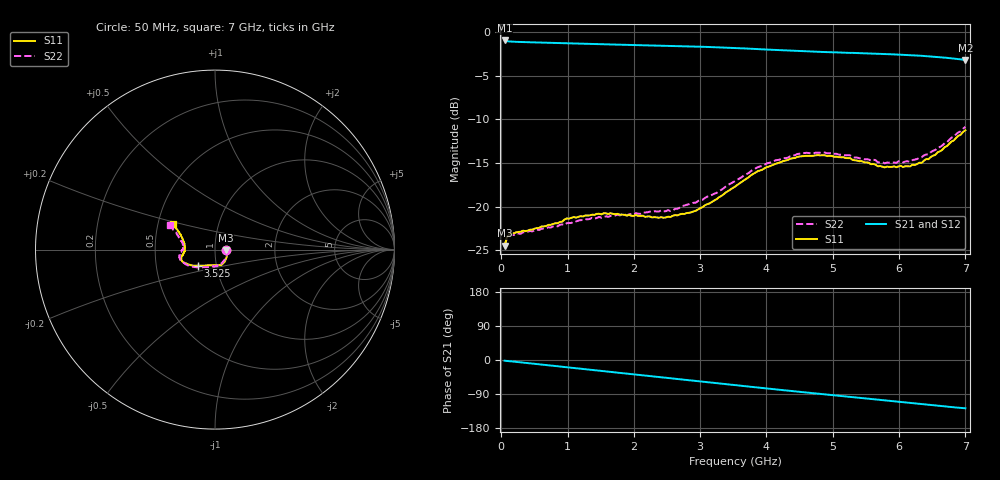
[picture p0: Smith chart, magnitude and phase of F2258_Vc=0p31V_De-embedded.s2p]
! Integrated Device Technology
! Corporate Headquarters
! 6024 Silver Creek Valley Road
! San Jose, CA 95138  USA
! Phone:  1-408-284-8200
! Toll Free:  1-800-223-1366
! Webpage:  http://www.idt.com/
! Timing and RF Division
! 515 Groton Road, Suite 102
! Westford, MA 01886-6024
! Device:  F2258
! Description: Voltage Variable RF Attenuator
! Frequency:  50.0 -  6000.00 MHz
! Package:  3x3 mm Thin QFN Plastic Package: 16 pin
! Ports:  2 RF, 2 DC
!  Pin  1  = NC
!  Pin  2  = NC
!  Pin  3  = RF2  = Port 2
!  Pin  4  = GND
!  Pin  5  = Vdd
!  Pin  6  = NC
!  Pin  7  = VCTRL
!  Pin  8  = NC
!  Pin  9  = GND
!  Pin 10  = RF1  = Port 1
!  Pin 11  = NC
!  Pin 12  = NC
!  Pin 13  = NC
!  Pin 14  = NC
!  Pin 15  = NC
!  Pin 16  = NC
! Vcntrl:  0.310 Volts
! Vdd:  +3.300 Volts
! Current:  1.086 mA
! Data:  The device was measured on a the F2258 evaluation board which has
!  individual transmission lines to the RF pins.  Data was collected
!  using a calibrated network analyzer.  The evaluation board was
!  de-embedded using a TRL calibration technique.
!  The reference plane is the edge of the package pin.
! Misc:  SN 10
!  Action Tracker AT0285
! Date Measured:  2014-12-10
! Date:  2016-01-13  MJV
! Note:
!  Integrated Device Technology supplies this data as a sample of measured
!  data at the package pin for this product.  Your particular data for this
!  product may vary.
!  Data was taken at 25 degrees C.
!  Integrated Device Technology reserves the right to change this data at anytime.
!Freq_(GHz)  S11M_(dB)  S11P_(deg)  S21M_(dB)  S21P_(deg)  S12M_(dB)  S12P_(deg)  S22M_(dB)  S22P_(deg)
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# GHz S dB R 50
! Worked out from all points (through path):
!   201 points, 50 MHz to 7 GHz, reference 50 ohm
!   highest |S21| = -0.98 dB at 50 MHz (marker M1); lowest = -3.2 dB at 7 GHz (marker M2)
!   group delay of S21, straight-line fit = 50.5 ps
!   lowest |S11| = -24.5 dB at 50 MHz (marker M3), VSWR 1.13, Z = 56.3 - j0.398 ohm
!   |S11| at or under -10 dB: start of sweep to end of sweep
!   |S22| runs from -24.5 to -10.9 dB; largest |S21 - S12| = 0.00045
!   S11 on the Smith chart (normalised r, x): 50 MHz: 1.13, -0.01; 3.525 GHz: 0.82, -0.15; 7 GHz: 0.60, +0.19
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0.05  -24.49 -3.4  -0.98 -1.9  -0.98 -1.9  -24.54 -3.0
0.08475  -23.53 -5.8  -1.06 -2.5  -1.06 -2.5  -23.61 -5.4
0.15425  -23.05 -9.0  -1.11 -3.6  -1.11 -3.6  -23.23 -9.3
0.71025  -22.11 -36.1  -1.25 -14.1  -1.25 -14.1  -22.38 -37.9
0.98825  -21.37 -49.8  -1.30 -19.3  -1.30 -19.3  -21.90 -53.8
1.2315  -21.14 -58.0  -1.35 -23.8  -1.35 -23.8  -21.55 -62.8
1.6485  -20.77 -69.5  -1.44 -31.4  -1.44 -31.4  -21.08 -75.9
2.37825  -21.29 -90.7  -1.57 -44.8  -1.57 -44.8  -20.56 -93.6
2.552  -21.19 -96.6  -1.60 -48.0  -1.60 -48.0  -20.52 -98.9
2.93425  -20.49 -113.3  -1.68 -55.1  -1.68 -55.1  -19.55 -112.4
3.525  -17.72 -136.5  -1.85 -66.2  -1.85 -66.2  -17.09 -135.1
3.76825  -16.41 -143.9  -1.93 -70.8  -1.94 -70.8  -15.92 -143.6
4.0115  -15.47 -150.4  -2.02 -75.2  -2.03 -75.2  -15.04 -150.6
4.46325  -14.32 -158.9  -2.19 -83.4  -2.19 -83.4  -14.00 -161.8
4.7065  -14.19 -162.2  -2.26 -87.7  -2.26 -87.7  -13.90 -166.0
5.2625  -14.47 -169.1  -2.41 -97.4  -2.41 -97.4  -14.14 -174.1
5.6795  -15.40 -175.8  -2.49 -104.6  -2.50 -104.6  -14.94 -179.5
5.85325  -15.47 -180.0  -2.55 -107.8  -2.55 -107.8  -14.98 175.8
6.166  -15.41 172.1  -2.65 -113.4  -2.66 -113.4  -14.89 169.9
6.33975  -15.00 165.7  -2.74 -116.5  -2.74 -116.5  -14.35 165.5
6.722  -13.08 153.9  -2.97 -123.1  -2.97 -123.1  -12.66 156.5
7  -11.26 148.4  -3.22 -127.4  -3.22 -127.4  -10.88 151.5
